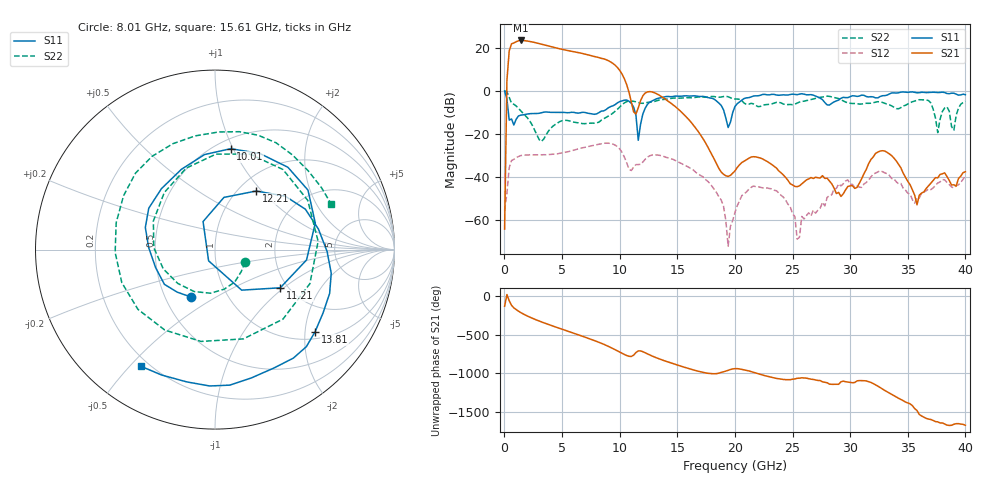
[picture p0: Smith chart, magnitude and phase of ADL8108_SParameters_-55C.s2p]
! Analog Devices, Inc.
! Device:	ADL8108 SN8565
! Description:	"GaAs, pHEMT, MMIC, Low Noise Amplifier,1.5 GHz to 6 GHz"
! Conditions:	Vdd = 5.0 V
!		Idq = 90 mA
!  Rbias = 1270 Ohm
!		Pin = -25 dBm
!		Operating Temperature = -55 C (at package bottom)
! Board loss de-embedded from S21 magnitude.  All other RF measurements reference to RF coaxial connector.
! Frequency (GHz)	S11_Mag (dB)	S11_Phase (deg)	S21_Mag (dB)	S21_Phase (deg)	S12_Mag (dB)	S12_Phase (deg)	S22_Mag (dB)	S22_Phase (deg)
#  GHZ  S  DB  R 50
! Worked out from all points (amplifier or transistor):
!   201 points, 10 MHz to 40 GHz, reference 50 ohm
!   highest |S21| = 23.4 dB at 1.41 GHz (marker M1)
!   |S21| within 3 dB of that: 520.7 MHz to 4.143 GHz (3.622 GHz wide, 155 % of centre)
!   unconditionally stable (mu >= 1): 44.47 MHz to end of sweep
!   at 6.61 GHz: K = 1.35, MAG = 18.5 dB, |S12| = -26.5 dB
!   at 20 GHz: K = 10839.22, MAG = -33.8 dB, |S12| = -56.3 dB
!   at 40 GHz: K = 732.89, MAG = -30.7 dB, |S12| = -39.2 dB
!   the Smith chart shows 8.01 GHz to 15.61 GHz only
!   S11 on the Smith chart (normalised r, x): 8.01 GHz: 0.67, -0.39; 10.01 GHz: 0.59, +0.98; 11.21 GHz: 1.83, -0.95; 12.21 GHz: 1.20, +0.93; 13.81 GHz: 1.18, -2.26; 15.61 GHz: 0.17, -0.54
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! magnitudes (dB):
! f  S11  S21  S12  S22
! 10 MHz  0.0  -64.0  -55.3  0.0
! 210 MHz  -3.7  4.8  -47.4  -0.4
! 410 MHz  -13.5  18.6  -35.5  -2.9
! 1.41 GHz  -11.2  23.4  -29.9  -9.2
! 6.81 GHz  -9.9  17.3  -26.3  -15.1
! 8.01 GHz  -10.6  15.7  -24.9  -14.8
! 10.01 GHz  -4.9  9.5  -26.9  -7.4
! 11.21 GHz  -7.5  -9.7  -35.2  -4.8
! 11.61 GHz  -22.8  -7.8  -34.1  -5.3
! 12.21 GHz  -8.0  -1.0  -31.6  -5.5
! 13.41 GHz  -3.3  -1.9  -29.7  -4.2
! 13.81 GHz  -2.8  -3.3  -30.3  -3.9
! 15.61 GHz  -2.3  -11.1  -34.4  -3.2
! 18.81 GHz  -6.7  -37.6  -50.5  -2.8
! 19.41 GHz  -16.9  -39.6  -71.9  -2.7
! 20.2 GHz  -5.9  -35.4  -53.2  -3.7
! 25.4 GHz  -1.7  -44.3  -68.7  -5.6
! 26.8 GHz  -1.9  -40.6  -55.2  -3.7
! 33.4 GHz  -1.4  -29.1  -39.1  -6.4
! 35.8 GHz  -0.8  -52.7  -49.3  -4.3
! 37.6 GHz  -0.7  -40.2  -42.7  -19.3
! 40 GHz  -1.7  -37.4  -39.2  -4.7
